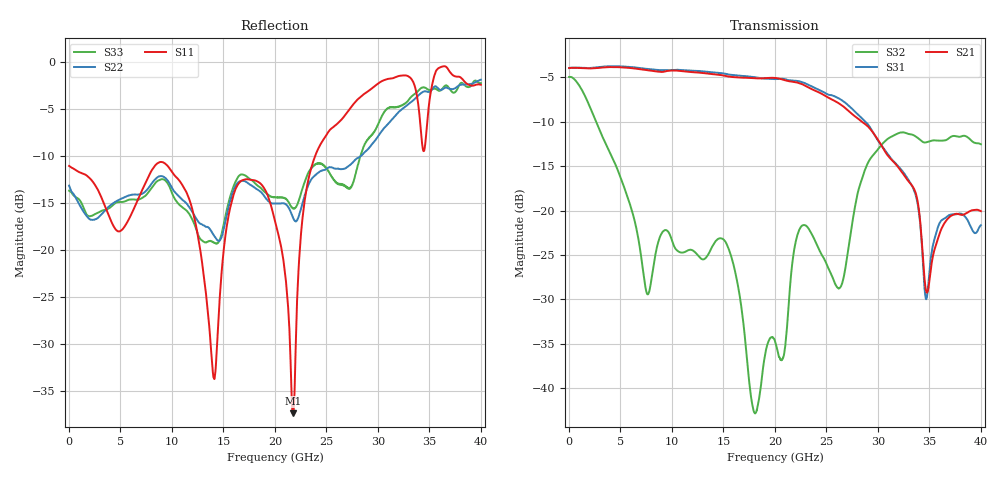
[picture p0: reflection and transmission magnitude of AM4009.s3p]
! AWR Design Environment (10030) Mon Oct 18 10:08:56 2021
! Document = 'Temporary_AM4009_RAW'
! nPorts: 3, nXvals: 6401
# GHz S RI R 50
!Freq ReS11 ImS11 ReS12 ImS12 ReS13 ImS13
!	ReS21 ImS21 ReS22 ImS22 ReS23 ImS23
!	ReS31 ImS31 ReS32 ImS32 ReS33 ImS33
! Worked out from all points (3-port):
!   6401 points, 10 MHz to 40 GHz, reference 50 ohm
!   strongest paths, dB at 10 MHz, 10.01 GHz, 20 GHz, 30 GHz, 40 GHz:
!     S21: -3.9, -4.2, -5.1, -12.0, -20.1
!     S31: -4.0, -4.2, -5.2, -12.1, -21.7
!     S32: -5.0, -23.4, -34.7, -13.1, -12.5
!   lowest |S11| = -37.4 dB at 21.72 GHz (marker M1), VSWR 1.03, Z = 51.3 - j0.548 ohm
!   |S11| at or under -10 dB: start of sweep to 23.92 GHz
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0.01  -0.2789 0.00271  0.6325 -0.0295  0.6342 -0.0233
      0.6345 -0.0276  -0.2185 0.0179  0.5816 -0.0321
      0.6338 -0.0148  0.5647 -0.0218  -0.2053 0.0164
5.65234  0.0836 -0.1124  -0.6331 -0.0859  -0.6408 -0.0634
         -0.631 -0.086  -0.1141 -0.1555  -0.1161 0.0332
         -0.6422 -0.063  -0.1161 0.0331  -0.0933 -0.1575
11.4634  -0.0509 0.1921  0.5998 0.0932  0.6102 0.0389
         0.5987 0.0919  -0.0848 0.1529  0.0186 0.0561
         0.6139 0.041  0.0184 0.0563  -0.0816 0.1383
14.0752  -0.00822 0.0191  0.165 -0.5628  0.1044 -0.5883
         0.1673 -0.561  -0.0331 0.1146  0.0593 -0.0263
         0.1043 -0.59  0.0597 -0.0263  -0.0559 0.0941
20.005  0.1008 -0.0998  -0.0331 0.5499  0.0606 0.5516
        -0.0326 0.5571  0.1282 0.1212  -0.0153 -0.00961
        0.0622 0.5465  -0.0157 -0.00962  0.0718 0.1757
21.7233  0.0124 -0.00535  0.4436 0.2827  0.503 0.1954
         0.4504 0.282  0.1376 0.0591  -0.044 -0.0286
         0.5026 0.1955  -0.0442 -0.0284  0.0967 0.1347
24.0977  0.3177 -0.1057  0.2664 -0.3792  0.1755 -0.4554
         0.269 -0.3824  0.2539 -0.00837  0.0272 0.0582
         0.169 -0.4529  0.0271 0.0577  0.2619 0.1165
30.2962  -0.7731 0.1183  0.0616 0.2159  0.1633 0.1743
         0.0678 0.2252  0.0169 0.4213  0.1785 0.1529
         0.1554 0.1755  0.175 0.1529  0.031 0.5021
35.6011  0.3677 0.7993  0.0476 -0.0393  0.0189 -0.0684
         0.041 -0.0479  0.2981 -0.676  -0.1469 -0.209
         0.0288 -0.0669  -0.1421 -0.2033  0.445 -0.5627
40  0.614 -0.436  -0.0916 0.0657  -0.0743 -0.00394
    -0.0804 0.058  -0.6636 -0.4473  -0.1525 0.1744
    -0.0827 0.00198  -0.1455 0.1859  -0.6136 -0.4619
